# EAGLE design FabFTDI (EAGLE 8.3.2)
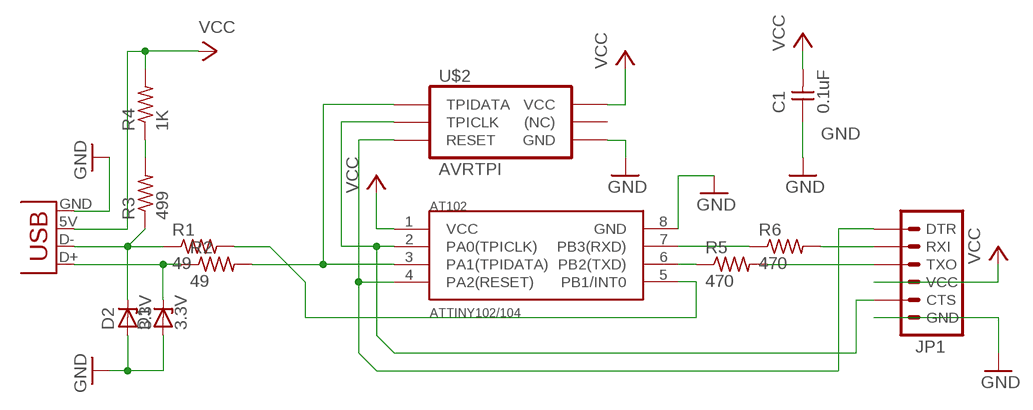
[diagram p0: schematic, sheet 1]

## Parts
C1  0.1uF  UNPOLARIZED_CAPACITOR1206  [1206]
D1  3.3V  ZENER_DIODESOD123  [SOD123]
D2  3.3V  ZENER_DIODESOD123  [SOD123]
JP1  FTDI_CONNECTORSMD  [1X06-SMD]
JP2  USBPCB  [USB_PCB]
R1  49  RESISTOR1206  [1206]
R2  49  RESISTOR1206  [1206]
R3  499  RESISTOR1206  [1206]
R4  1K  RESISTOR1206  [1206]
R5  470  RESISTOR1206  [1206]
R6  470  RESISTOR1206  [1206]
U$1  ATTINY102/104  [SOIC8]
U$2  AVRTPISMD  [2X03SMD]

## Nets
GND: C1.1 D1.ANODE D2.ANODE JP1.6(GND) JP2.GND U$1.8(GND) U$2.6(GND)
N$1: D1.CATHODE JP2.D+ R2.1
N$2: D2.CATHODE JP2.D- R1.1 R3.1
N$3: R1.2 U$1.5(PB1/INT0)
N$4: R2.2 U$1.3(PA1(TPIDATA)) U$2.1(TPIDATA)
N$5: R3.2 R4.1
N$7: JP1.2(RXI) R6.2
N$8: JP1.3(TXO) R5.2
N$9: JP1.1(DTR) U$1.4(PA2(RESET)) U$2.5(RESET)
N$10: R6.1 U$1.7(PB3(RXD))
N$11: R5.1 U$1.6(PB2(TXD))
N$13: JP1.5(CTS) U$1.2(PA0(TPICLK)) U$2.3(TPICLK)
VCC: C1.2 JP1.4(VCC) JP2.5V(VBUS) R4.2 U$1.1(VCC) U$2.2(VCC)
Unconnected: U$2.4((NC))

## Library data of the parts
C1 = fabPatil:UNPOLARIZED_CAPACITOR: unpolarized_capacitor
D1 D2 = fabPatil:ZENER_DIODE: zener diode
JP1 = fabPatil:FTDI_CONNECTOR: FTDI connector smd
JP2 = fabPatil:USB: USB Connector Connector for USB-microB (orAB), USB-mini, and USB-PCB. For USB-micro use Digikey Part# 609-4052-1-ND (typeB) or 609-4052-1-ND (typeAB).
R1-R6 = fabPatil:RESISTOR
U$1 = fabPatil:ATTINY102/104: ATTINY102/104 Device for ATTINY102/104
U$2 = fabPatil:AVRTPI: ATMEL-ICE TPI Connector SMD This is a TPI programming connector to program Atiny102/104 micro-controllers prashant.patil@cba.mit.edu

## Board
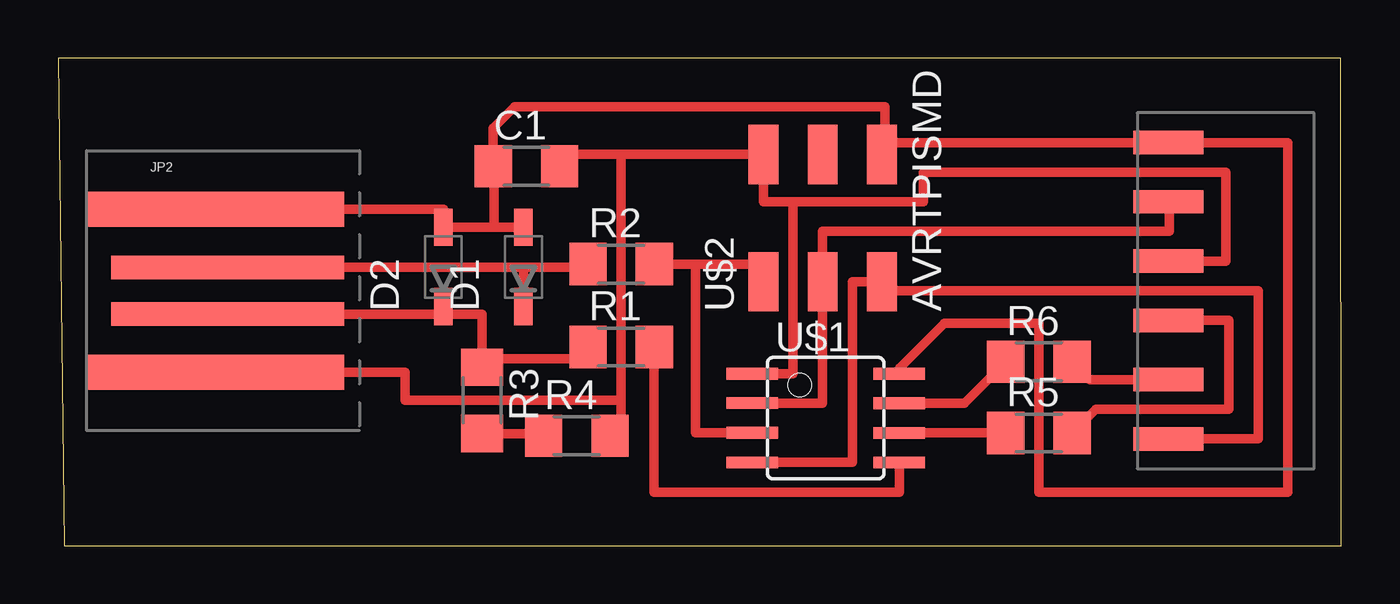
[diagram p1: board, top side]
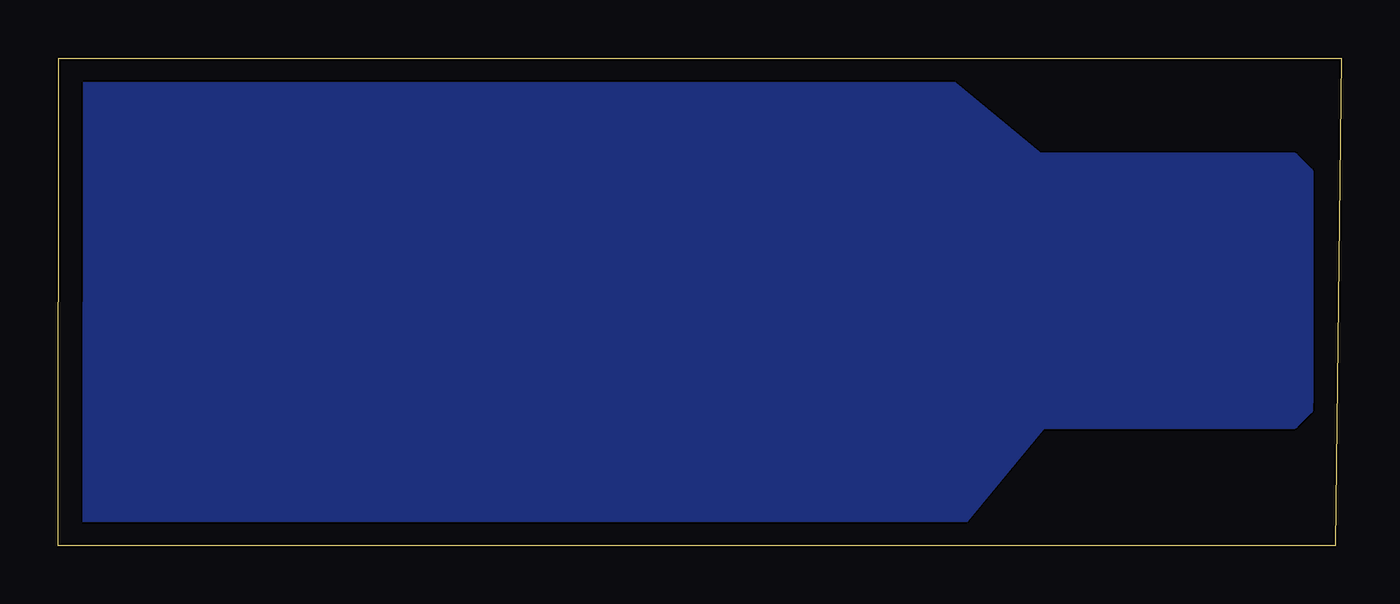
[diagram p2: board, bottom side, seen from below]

Size 54.99 x 20.88 mm. Coordinates in mm from the lower left corner, seen from the top.
Outline: 0.25,0 54.99,0 54.97,20.88 0,20.88 0.25,0
Copper layers (1*16): Top 0.035mm / dielectric 1.5mm / Bottom 0.035mm
Design rules "Patil": minimum track width 10mil, minimum drill 24mil, track to track 16mil, track to pad 16mil, pad to pad 16mil, via to via 16mil, smd to smd 16mil, copper to edge 40mil, drill to drill 8mil, minimum pad ring 10mil, minimum via ring 8mil, stop-mask expansion 4mil, vias tented up to drill 0mil, thermal gap 10mil

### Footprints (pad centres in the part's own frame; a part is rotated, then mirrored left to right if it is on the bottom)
1206 = smd 1.6 x 1.803: 1 -1.422,0; 2 1.422,0
SOD123 = smd 1.6 x 0.8: ANODE 1.7,0; CATHODE -1.7,0
1X06-SMD = smd 1 x 3: 1 -6.35,-1.35; 2 -3.81,-1.35; 3 -1.27,-1.35; 4 1.27,-1.35; 5 3.81,-1.35; 6 6.35,-1.35
USB_PCB = smd 11 x 1.5: 5V 1.55,-3.5; GND 1.55,3.5 | smd 10 x 1: D+ 2.05,1; D- 2.05,-1
SOIC8 = smd 0.5 x 2.2: 1 -1.905,-3.154; 2 -0.645,-3.154; 3 0.625,-3.154; 4 1.895,-3.154; 5 1.905,3.154; 6 0.635,3.154; 7 -0.635,3.154; 8 -1.905,3.154
2X03SMD = smd 2.54 x 1.27: 1 -2.54,2.54; 2 2.92,2.54; 3 -2.54,0; 4 2.92,0; 5 -2.54,-2.54; 6 2.92,-2.54

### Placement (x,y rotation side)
C1  20.07,16.26 0 top
D1  19.94,11.94 90 top
D2  16.51,11.94 90 top
JP1  46.23,10.92 90 top
JP2  5.21,10.92 0 top
R1  24.13,8.51 0 top
R2  24.13,12.06 0 top
R3  18.16,6.22 270 top
R4  22.23,4.7 0 top
R5  42.04,4.83 0 top
R6  42.04,7.87 0 top
U$1  32.89,5.46 270 top
U$2  32.77,13.84 90 top

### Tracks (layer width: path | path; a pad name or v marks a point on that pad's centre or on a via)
GND
  Top 0.406: JP2.GND 16.51,14.42 D2.ANODE 18.67,13.64 | 18.67,13.64 D1.ANODE | U$2.6 35.43,16.76 35.43,17.27 | 35.43,17.27 35.43,18.8 19.56,18.8 18.64,17.88 C1.1 18.67,16 18.67,13.64 | 35.43,17.27 JP1.6 52.7,17.27 52.7,2.29 42.04,2.29 42.04,9.53 37.97,9.53 36.05,7.6 U$1.8 36.83,7.37
N$1
  Top 0.406: 9.81,11.68 JP2.D+ 19.94,11.92 | 19.94,11.92 D1.CATHODE | 19.94,11.92 22.71,11.92 R2.1
N$2
  Top 0.406: JP2.D- 9.59,9.91 16.51,9.91 | 16.51,9.91 D2.CATHODE | 18.16,8 R3.1 | 18.16,8 18.16,9.91 16.51,9.91 | R1.1 22.71,8 18.16,8
N$3
  Top 0.406: U$1.5 36.05,2.29 25.53,2.29 25.53,8.51 R1.2
N$4
  Top 0.406: 27.3,12.06 30.23,12.06 U$2.1 | 27.3,12.06 27.3,4.84 U$1.3 | 27.3,12.06 R2.2
N$5
  Top 0.406: 18.16,4.7 R3.2 20.8,4.8 R4.1
N$6
  pour Bottom (no thermals): 1.4,16 2.03,16.64 12.95,16.64 17.27,20.19 53.09,20.19 54.1,19.81 arc-3 54.1,1.27 52.83,0.89 16.38,0.89 12.83,5.21 2.03,5.21 1.4,5.84
N$7
  Top 0.406: JP1.2 44.22,7.11 R6.2
N$8
  Top 0.406: R5.2 44.47,5.84 50.16,5.84 50.16,9.65 JP1.3
N$9
  Top 0.406: U$1.4 34.04,3.57 34.04,11.3 U$2.5 35.05,11.3 35.05,10.92 51.43,10.92 51.43,4.57 JP1.1
N$10
  Top 0.406: U$1.7 38.84,6.1 R6.1
N$11
  Top 0.406: U$1.6 R5.1
N$13
  Top 0.406: U$1.2 32.77,6.11 U$2.3 32.77,13.46 47.62,13.46 47.62,14.73 JP1.5
VCC
  Top 0.406: 29.72,7.37 U$1.1 31.5,7.37 31.5,14.73 | 30.23,16.89 U$2.2 | JP1.4 50.04,12.19 50.04,16 37.08,16 37.08,14.73 31.5,14.73 | 22,16.76 C1.2 21.49,16.76 24.13,16.76 | 24.13,16.76 U$2.2 | JP2.5V 14.86,7.42 14.86,6.22 24.13,6.22 | 24.13,16.76 24.13,6.22 | 24.13,6.22 24.13,4.7 R4.2 | U$2.2 30.23,14.73 31.5,14.73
